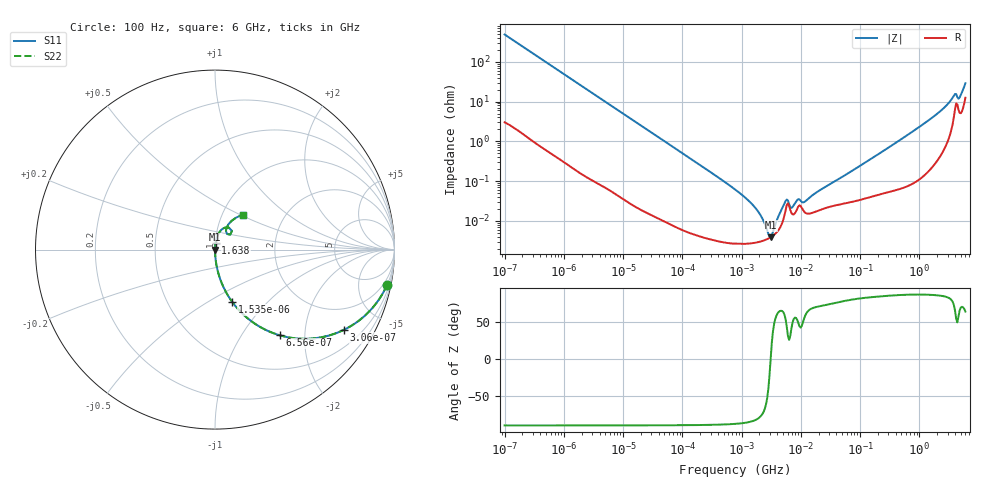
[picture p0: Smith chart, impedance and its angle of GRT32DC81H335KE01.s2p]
!Murata Part Number: GRT32DC81H335KE01
!These Parameters are Measured in Series Mode Connection
!Data Generated on Jun 19, 2026
!  o--ll--o
!Port1  Port2
!  o------o
!Operation Temp=25[degC], DC Bias Voltage=0[V]
!Freq. Start=100[Hz] Stop=6[GHz] 401[Steps]
# Hz S RI R 50
!Freq.(Hz) S11(Real) S11(Imag) S21(Real) S21(Imag) S12(Real) S12(Imag) S22(Real) S22(Imag)
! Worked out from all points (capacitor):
!   401 points, 100 Hz to 6 GHz, reference 50 ohm
!   read as one part in series: C = 3.25 uF near 109 Hz
!   lowest |Z| = 3.85 mohm at 3.104 MHz (marker M1)
!   series resonance near 3.091 MHz, so ESL is about 810 pH
!   S11 on the Smith chart (normalised r, x): 100 Hz: 1.06, -9.76; 306 Hz: 1.02, -3.20; 656 Hz: 1.01, -1.50; 1.535 kHz: 1.00, -0.64; 1.638 GHz: 1.00, +0.08; 6 GHz: 1.25, +0.52
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100  0.9586 -0.1961  0.0414 0.1961  0.0414 0.1961  0.9586 -0.1961
306  0.7185 -0.4467  0.2815 0.4467  0.2815 0.4467  0.7185 -0.4467
656  0.3612 -0.4773  0.6388 0.4773  0.6388 0.4773  0.3612 -0.4773
1535  0.0952 -0.2905  0.9048 0.2905  0.9048 0.2905  0.0952 -0.2905
2008  0.0583 -0.2314  0.9417 0.2314  0.9417 0.2314  0.0583 -0.2314
6728  0.00593 -0.0733  0.9941 0.0733  0.9941 0.0733  0.00593 -0.0733
40335  0.000266 -0.0124  0.9997 0.0124  0.9997 0.0124  0.000266 -0.0124
774597  2.68e-05 -0.000615  1 0.000615  1 0.000615  2.68e-05 -0.000615
1449809  2.71e-05 -0.000276  1 0.000276  1 0.000276  2.71e-05 -0.000276
2372521  3.18e-05 -9.04e-05  1 9.04e-05  1 9.04e-05  3.18e-05 -9.04e-05
3103719  3.85e-05 1.4e-06  1 -1.4e-06  1 -1.4e-06  3.85e-05 1.4e-06
3882480  5.05e-05 8.37e-05  0.9999 -8.37e-05  0.9999 -8.37e-05  5.05e-05 8.37e-05
5554849  0.000189 0.000254  0.9998 -0.000254  0.9998 -0.000254  0.000189 0.000254
7266822  0.000145 0.00017  0.9999 -0.00017  0.9999 -0.00017  0.000145 0.00017
8692127  0.0002 0.000266  0.9998 -0.000266  0.9998 -0.000266  0.0002 0.000266
1.137099e7  0.000169 0.000241  0.9998 -0.000241  0.9998 -0.000241  0.000169 0.000241
1.555665e7  0.000158 0.000404  0.9998 -0.000404  0.9998 -0.000404  0.000158 0.000404
3.124326e8  0.000582 0.00714  0.9994 -0.00714  0.9994 -0.00714  0.000582 0.00714
1.637704e9  0.00369 0.0388  0.9963 -0.0388  0.9963 -0.0388  0.00369 0.0388
3.8344e9  0.0552 0.1224  0.9448 -0.1224  0.9448 -0.1224  0.0552 0.1224
4.796499e9  0.0608 0.1034  0.9392 -0.1034  0.9392 -0.1034  0.0608 0.1034
6e9  0.156 0.1949  0.844 -0.1949  0.844 -0.1949  0.156 0.1949
